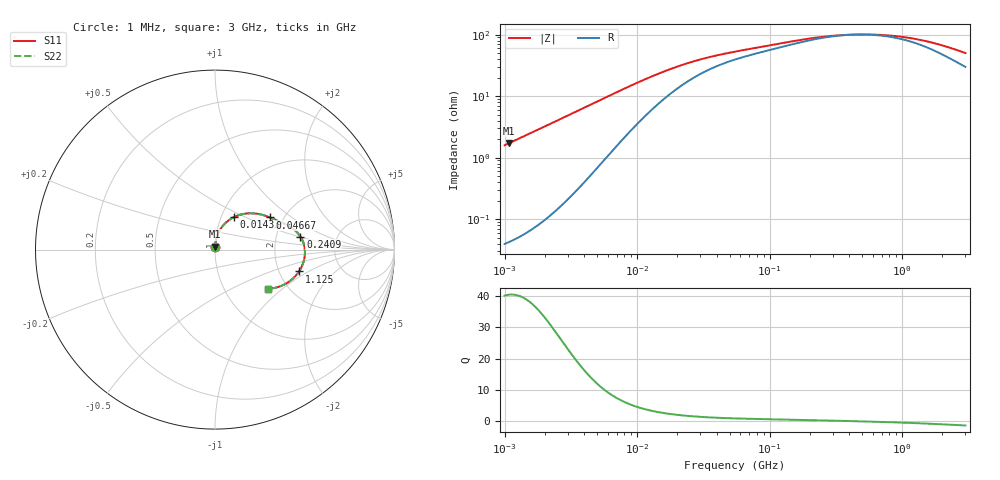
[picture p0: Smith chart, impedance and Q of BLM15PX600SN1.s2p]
! BLM15PX600SN1
# Hz S RI R 50
!Freq.(Hz) S11(Real) S11(Imag) S21(Real) S21(Imag) S12(Real) S12(Imag) S22(Real) S22(Imag)
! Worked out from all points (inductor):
!   401 points, 1 MHz to 3 GHz, reference 50 ohm
!   read as one part in series: L = 253 nH near 1.041 MHz
!   highest Q = 40.5 at 1.083 MHz (marker M1), where L = 253 nH
!   self-resonance near 451.9 MHz
!   S11 on the Smith chart (normalised r, x): 1 MHz: 1.00, +0.03; 14.33 MHz: 1.15, +0.43; 46.67 MHz: 1.70, +0.70; 240.9 MHz: 2.75, +0.52; 1.125 GHz: 2.57, -0.82; 3 GHz: 1.60, -0.81
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1000000  0.000648 0.0159  0.9994 -0.0159  0.9994 -0.0159  0.000648 0.0159
1083356  0.000722 0.0172  0.9993 -0.0172  0.9993 -0.0172  0.000722 0.0172
2182827  0.00234 0.0348  0.9977 -0.0348  0.9977 -0.0348  0.00234 0.0348
3823119  0.00737 0.0613  0.9926 -0.0613  0.9926 -0.0613  0.00737 0.0613
7858845  0.0352 0.1214  0.9648 -0.1214  0.9648 -0.1214  0.0352 0.1214
1.082539e7  0.0658 0.1549  0.9342 -0.1549  0.9342 -0.1549  0.0658 0.1549
1.432659e7  0.1053 0.1809  0.8947 -0.1809  0.8947 -0.1809  0.1053 0.1809
1.461624e7  0.1086 0.1825  0.8914 -0.1825  0.8914 -0.1825  0.1086 0.1825
1.896016e7  0.1543 0.1979  0.8457 -0.1979  0.8457 -0.1979  0.1543 0.1979
2.509235e7  0.2066 0.2023  0.7934 -0.2023  0.7934 -0.2023  0.2066 0.2023
3.320783e7  0.2556 0.1956  0.7444 -0.1956  0.7444 -0.1956  0.2556 0.1956
4.666789e7  0.3055 0.1795  0.6945 -0.1795  0.6945 -0.1795  0.3055 0.1795
5.477226e7  0.3256 0.1711  0.6744 -0.1711  0.6744 -0.1711  0.3256 0.1711
1.244416e8  0.4158 0.1285  0.5842 -0.1285  0.5842 -0.1285  0.4158 0.1285
2.094008e8  0.4656 0.0867  0.5344 -0.0867  0.5344 -0.0867  0.4656 0.0867
2.408952e8  0.476 0.0725  0.524 -0.0725  0.524 -0.0725  0.476 0.0725
4.480278e8  0.5005 0.00106  0.4995 -0.00106  0.4995 -0.00106  0.5005 0.00106
8.005644e8  0.4913 -0.0743  0.5087 0.0743  0.5087 0.0743  0.4913 -0.0743
1.125055e9  0.4679 -0.122  0.5321 0.122  0.5321 0.122  0.4679 -0.122
1.855641e9  0.3992 -0.1874  0.6008 0.1874  0.6008 0.1874  0.3992 -0.1874
2.407135e9  0.3469 -0.2099  0.6531 0.2099  0.6531 0.2099  0.3469 -0.2099
3e9  0.2976 -0.2178  0.7024 0.2178  0.7024 0.2178  0.2976 -0.2178
